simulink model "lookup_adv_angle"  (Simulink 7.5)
settings: Solver=ode113  StartTime=0.0  StopTime=2  MaxStep=1e-4  MinStep=1e-5  RelTol=1e-5
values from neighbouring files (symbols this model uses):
  B = 0.0001    [adv1.m]    (also in adv1_plot_eaia.m; adv1_plot_te_speed.m; lookup01_plot.m; NEW_VAR .m)
  BV = 24    [adv1.m]    (also in adv1_plot_eaia.m; adv1_plot_te_speed.m; lookup01_plot.m; NEW_VAR .m)
  J = .0001    (= 0.0001)    [adv1.m]    (also in adv1_plot_eaia.m; adv1_plot_te_speed.m; lookup01_plot.m; NEW_VAR .m)
  kw = 0.0445    [adv1.m]    (also in adv1_plot_eaia.m; adv1_plot_te_speed.m; lookup01_plot.m = 0.0365; NEW_VAR .m)
  L = .00192    (= 0.00192)    [adv1.m]    (also in adv1_plot_eaia.m; adv1_plot_te_speed.m; lookup01_plot.m; NEW_VAR .m)
  P = 4    [adv1.m]    (also in adv1_plot_eaia.m; adv1_plot_te_speed.m; lookup01_plot.m; NEW_VAR .m)
  R = 1.5    [adv1.m]    (also in adv1_plot_eaia.m; adv1_plot_te_speed.m; lookup01_plot.m; NEW_VAR .m)
  T0 = 0.0001    [adv1.m]    (also in adv1_plot_eaia.m; adv1_plot_te_speed.m; lookup01_plot.m; NEW_VAR .m)
  W0 = 2    [adv1.m]    (also in adv1_plot_eaia.m; adv1_plot_te_speed.m; lookup01_plot.m; NEW_VAR .m)
libraries: simulink x1

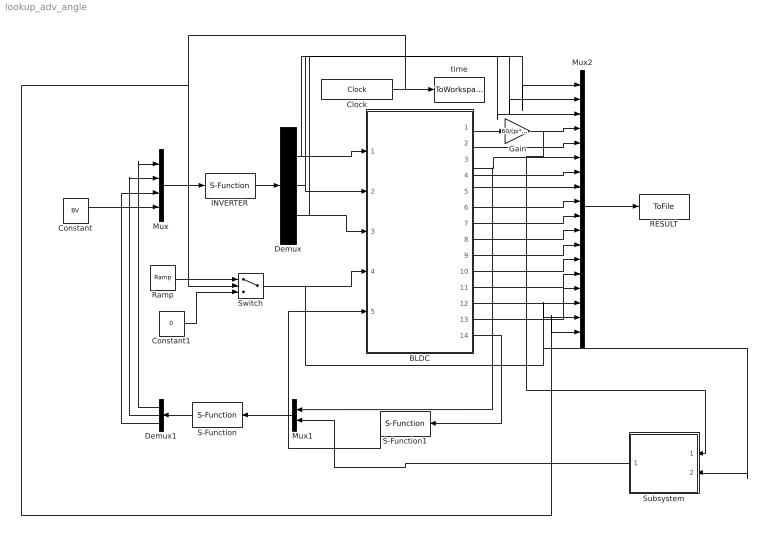
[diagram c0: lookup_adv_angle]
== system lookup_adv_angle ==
  BLDC : Subsystem
  Clock : Clock
  Constant : Constant  Value=BV  OutDataType=fixdt(1, 16)  OutScaling=2^0
  Constant1 : Constant  Value=0  OutDataType=fixdt(1, 16)  OutScaling=2^0
  Demux : Demux  Outputs=3
  Demux1 : Demux  Outputs=3
  Gain : Gain  Gain=60/(pi*P)  ParameterDataType=fixdt(1, 16)  ParameterScaling=2^0  OutDataType=fixdt(1, 16)  OutScaling=2^0
  INVERTER : S-Function  FunctionName=inverter  Parameters=vmax  EnableBusSupport=off  mask{vmax=50}
      mask prompts: vmax "maximum dc bus"
  Mux : Mux
  Mux1 : Mux  Inputs=2
  Mux2 : Mux  Inputs=18
  RESULT : ToFile  Filename=bldc_advangle
  Ramp : simulink/Sources/Ramp  SystemSampleTime=-1  slope=0.5  start=1  X0=0
  S-Function : S-Function  FunctionName=BLDC_adv_2in  Parameters=angle  EnableBusSupport=off  mask{angle=0}
      mask prompts: angle "advance  angle"
  S-Function1 : S-Function  FunctionName=sam_adv_ktc  Parameters=R,L,J,P,kw  EnableBusSupport=off
  Subsystem : Subsystem
  Switch : Switch  Threshold=1  OutDataType=fixdt(1, 16)  OutScaling=2^0
  time : ToWorkspace  VariableName=time  SampleTime=-1  SaveFormat=Array
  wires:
  INVERTER/1 -> Demux/1
  Mux/1 -> INVERTER/1
  BLDC/1(W) -> Gain/1
  Clock/1 -> time/1, Switch/2, Mux2/18
  S-Function/1 -> Demux1/1
  Constant/1 -> Mux/4
  BLDC/14(outadv) -> S-Function1/1
  Mux1/1 -> S-Function/1
  BLDC/3(Phi) -> Mux1/1, Mux2/6
  Switch/1 -> BLDC/4(Tload), Mux2/17, Subsystem/2(load)
  S-Function1/1 -> BLDC/5(inadv)
  Demux/1 -> BLDC/1(Va), Mux2/1
  Demux/2 -> BLDC/2(Vb), Mux2/2
  Demux/3 -> BLDC/3(Vc), Mux2/3
  Demux1/1 -> Mux/1
  Demux1/2 -> Mux/2
  Demux1/3 -> Mux/3
  Subsystem/1(angle) -> Mux1/2
  Gain/1 -> Mux2/4, Subsystem/1(speed)
  BLDC/2(Te) -> Mux2/5
  BLDC/4(HA) -> Mux2/7
  BLDC/5(HB) -> Mux2/8
  BLDC/6(HC) -> Mux2/9
  BLDC/7(ea) -> Mux2/10
  BLDC/8(eb) -> Mux2/11
  BLDC/9(ec) -> Mux2/12
  BLDC/10(theta) -> Mux2/13
  BLDC/11(ic) -> Mux2/14
  BLDC/12(ib) -> Mux2/15
  BLDC/13(ia) -> Mux2/16
  Mux2/1 -> RESULT/1
  Constant1/1 -> Switch/3
  Ramp/1 -> Switch/1

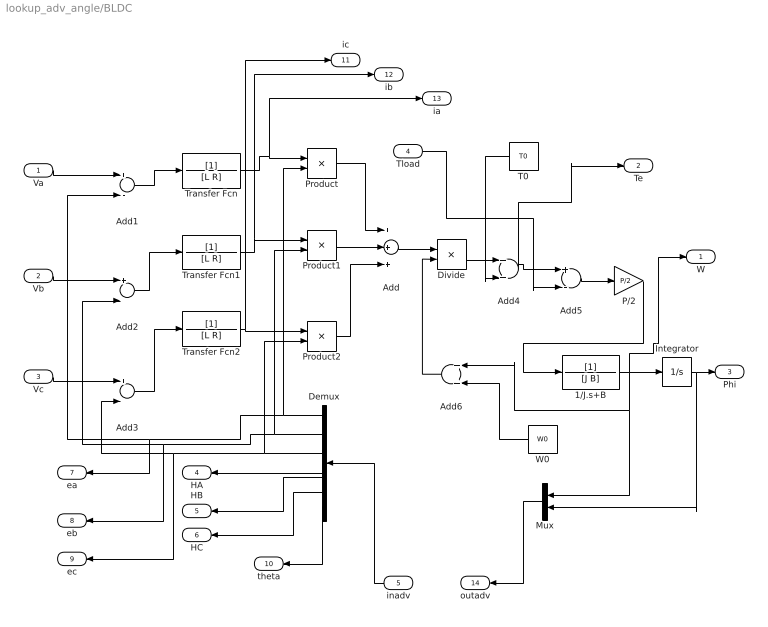
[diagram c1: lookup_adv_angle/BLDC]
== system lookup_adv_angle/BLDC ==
  Va : Inport  OutDataType=fixdt(1, 16)  OutScaling=2^0
  Vb : Inport  Port=2  OutDataType=fixdt(1, 16)  OutScaling=2^0
  Vc : Inport  Port=3  OutDataType=fixdt(1, 16)  OutScaling=2^0
  Tload : Inport  Port=4  OutDataType=fixdt(1, 16)  OutScaling=2^0
  inadv : Inport  Port=5  OutDataType=fixdt(1, 16)  OutScaling=2^0
  1/J.s+B : TransferFcn  Denominator=[J B]
  Add : Sum  Inputs=+++  OutDataType=fixdt(1, 16)  OutScaling=2^-10
  Add{1..3,5} (4 alike) : Sum  Inputs=+-  OutDataType=fixdt(1, 16)  OutScaling=2^-10
  Add4 : Sum  OutDataType=fixdt(1, 16)  OutScaling=2^-10
  Add6 : Sum  OutDataType=fixdt(1, 16)  OutScaling=2^-10
  Demux : Demux  Outputs=7
  Divide : Product  Inputs=*/  OutDataType=fixdt(1, 16)  OutScaling=2^-10
  Integrator : Integrator
  Mux : Mux  Inputs=2
  P/2 : Gain  Gain=P/2  ParameterDataType=fixdt(1, 16)  ParameterScaling=2^0  OutDataType=fixdt(1, 16)  OutScaling=2^0
  Product : Product  OutDataType=fixdt(1, 16)  OutScaling=2^0
  Product1 : Product  OutDataType=fixdt(1, 16)  OutScaling=2^0
  Product2 : Product  OutDataType=fixdt(1, 16)  OutScaling=2^0
  T0 : Constant  Value=T0  OutDataType=fixdt(1, 16)  OutScaling=2^0
  Transfer Fcn : TransferFcn  Denominator=[L R]
  Transfer Fcn1 : TransferFcn  Denominator=[L R]
  Transfer Fcn2 : TransferFcn  Denominator=[L R]
  W0 : Constant  Value=W0  OutDataType=fixdt(1, 16)  OutScaling=2^0
  W : Outport  OutDataType=fixdt(1, 16)  OutScaling=2^0
  Te : Outport  Port=2  OutDataType=fixdt(1, 16)  OutScaling=2^0
  Phi : Outport  Port=3  OutDataType=fixdt(1, 16)  OutScaling=2^0
  HA : Outport  Port=4  OutDataType=fixdt(1, 16)  OutScaling=2^0
  HB : Outport  Port=5  OutDataType=fixdt(1, 16)  OutScaling=2^0
  HC : Outport  Port=6  OutDataType=fixdt(1, 16)  OutScaling=2^0
  ea : Outport  Port=7  OutDataType=fixdt(1, 16)  OutScaling=2^0
  eb : Outport  Port=8  OutDataType=fixdt(1, 16)  OutScaling=2^0
  ec : Outport  Port=9  OutDataType=fixdt(1, 16)  OutScaling=2^0
  theta : Outport  Port=10  OutDataType=fixdt(1, 16)  OutScaling=2^0
  ic : Outport  Port=11  OutDataType=fixdt(1, 16)  OutScaling=2^0
  ib : Outport  Port=12  OutDataType=fixdt(1, 16)  OutScaling=2^0
  ia : Outport  Port=13  OutDataType=fixdt(1, 16)  OutScaling=2^0
  outadv : Outport  Port=14  OutDataType=fixdt(1, 16)  OutScaling=2^0
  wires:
  Add1/1 -> Transfer Fcn/1
  Add2/1 -> Transfer Fcn1/1
  Add3/1 -> Transfer Fcn2/1
  Transfer Fcn/1 -> Product/1, ia/1
  Transfer Fcn1/1 -> Product1/1, ib/1
  Transfer Fcn2/1 -> Product2/1, ic/1
  Demux/1 -> Add1/2, ea/1, Product/2
  Demux/2 -> Product1/2, Add2/2, eb/1
  Va/1 -> Add1/1
  Vb/1 -> Add2/1
  Vc/1 -> Add3/1
  Demux/3 -> Product2/2, Add3/2, ec/1
  Product/1 -> Add/1
  Product1/1 -> Add/2
  Product2/1 -> Add/3
  Add/1 -> Divide/1
  Add5/1 -> P/2/1
  Divide/1 -> Add4/1
  T0/1 -> Add4/2
  Add4/1 -> Add5/1, Te/1
  Tload/1 -> Add5/2
  P/2/1 -> 1/J.s+B/1
  1/J.s+B/1 -> Integrator/1, W/1, Add6/1, Mux/1
  Add6/1 -> Divide/2
  W0/1 -> Add6/2
  Integrator/1 -> Phi/1, Mux/2
  Demux/4 -> HA/1
  Demux/5 -> HB/1
  Demux/6 -> HC/1
  Demux/7 -> theta/1
  inadv/1 -> Demux/1
  Mux/1 -> outadv/1

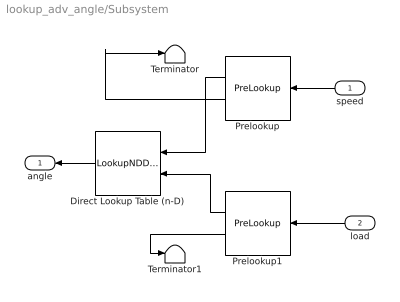
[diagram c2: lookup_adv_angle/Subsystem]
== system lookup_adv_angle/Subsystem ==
  speed : Inport  OutDataType=fixdt(1, 16)  OutScaling=2^0
  load : Inport  Port=2  OutDataType=fixdt(1, 16)  OutScaling=2^0
  Direct Lookup Table (n-D) : LookupNDDirect  Table=reshape([-0.5,-0.5,-0.55,-0.55,-0.1,-0.1,0.1,0.13,0.15,0.25,-0.5,-0.5,-0.55,-0.55,-0.1,-0.1,0.1,0.13,0.15,0.25,-0.5,-0.5,-0.55,-0.55,-0.1,-0.1,0.1,0.13,0.15,0.25,-0.5,-0.5,-0.55,-0.55,-0.1,-0.1,0.1,0.13,0.15,0.25,-0.5,-0.5,-0.55,-0.55,-0.1,-0.1,0.1,0.13,0.15,0.25,-0.55,-0.55,-0.55,-0.55,-0.1,-0.1,0.1,0.13,0.15,0.25,-0.55,-0.55,-0.55,-0.55,-0.55,-0.55,-0.55,-0.55,-0.55,-0.55,-0.55,-0.55,-0.55,-0.55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
  Prelookup : PreLookup  BreakpointsData=[1000:200:2800]  ProcessOutOfRangeInput=Linear extrapolation  IndexDataType=fixdt(1, 16)  FractionDataType=fixdt(1, 16)  FractionScaling=2^0
  Prelookup1 : PreLookup  BreakpointsData=[0.05:0.05:0.5]  ProcessOutOfRangeInput=Linear extrapolation  IndexDataType=fixdt(1, 16)  FractionDataType=fixdt(1, 16)  FractionScaling=2^0
  Terminator : Terminator
  Terminator1 : Terminator
  angle : Outport  OutDataType=fixdt(1, 16)  OutScaling=2^0
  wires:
  Prelookup1/1 -> Direct Lookup Table (n-D)/2
  Prelookup/1 -> Direct Lookup Table (n-D)/1
  speed/1 -> Prelookup/1
  load/1 -> Prelookup1/1
  Direct Lookup Table (n-D)/1 -> angle/1
  Prelookup/2 -> Terminator/1
  Prelookup1/2 -> Terminator1/1
